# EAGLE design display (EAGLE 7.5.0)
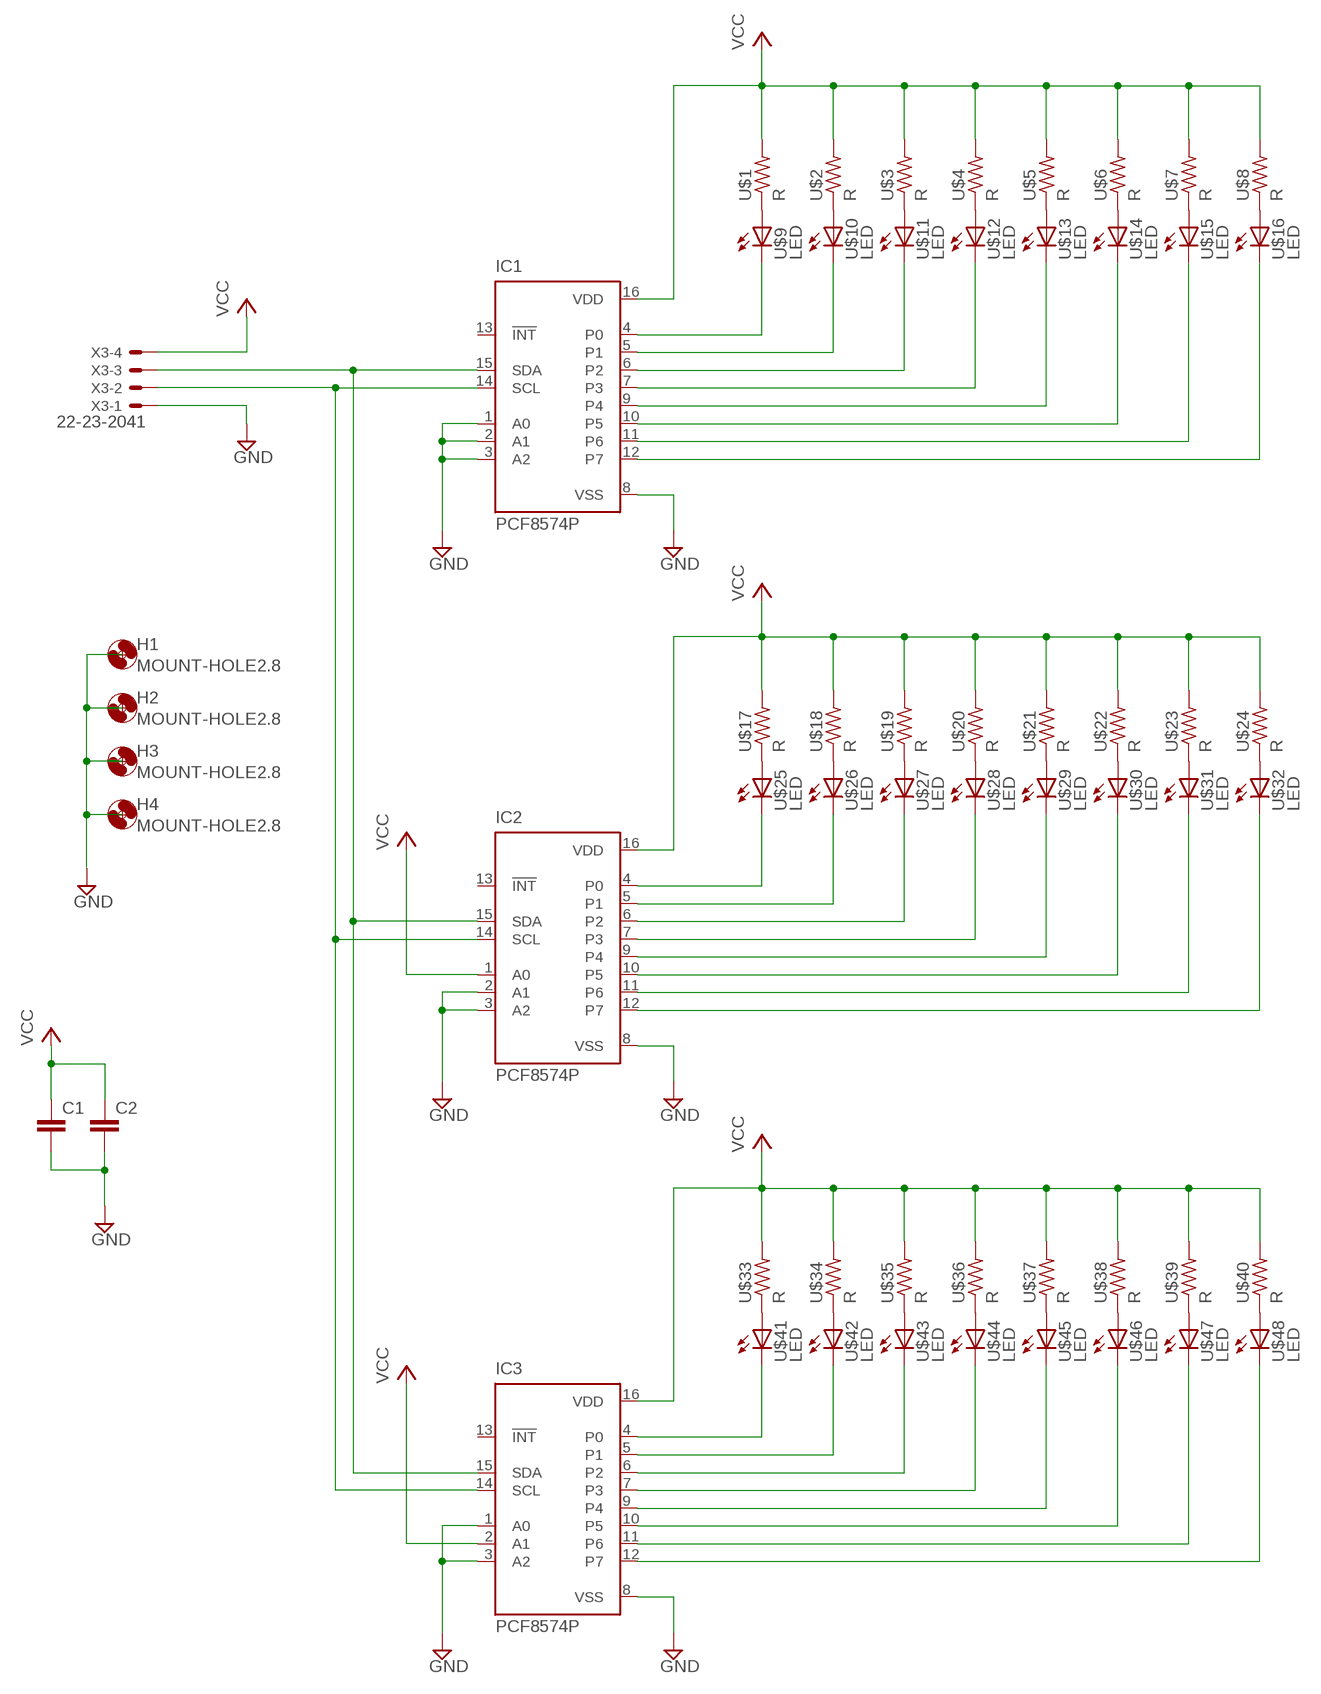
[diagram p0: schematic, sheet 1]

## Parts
C1  C-EU050-045X075  [C050-045X075]
C2  C-EU050-045X075  [C050-045X075]
H1  MOUNT-HOLE2.8  [2,8]
H2  MOUNT-HOLE2.8  [2,8]
H3  MOUNT-HOLE2.8  [2,8]
H4  MOUNT-HOLE2.8  [2,8]
IC1  PCF8574P  [DIL16]
IC2  PCF8574P  [DIL16]
IC3  PCF8574P  [DIL16]
U$1  R  [R]
U$2  R  [R]
U$3  R  [R]
U$4  R  [R]
U$5  R  [R]
U$6  R  [R]
U$7  R  [R]
U$8  R  [R]
U$9  LED  [LED]
U$10  LED  [LED]
U$11  LED  [LED]
U$12  LED  [LED]
U$13  LED  [LED]
U$14  LED  [LED]
U$15  LED  [LED]
U$16  LED  [LED]
U$17  R  [R]
U$18  R  [R]
U$19  R  [R]
U$20  R  [R]
U$21  R  [R]
U$22  R  [R]
U$23  R  [R]
U$24  R  [R]
U$25  LED  [LED]
U$26  LED  [LED]
U$27  LED  [LED]
U$28  LED  [LED]
U$29  LED  [LED]
U$30  LED  [LED]
U$31  LED  [LED]
U$32  LED  [LED]
U$33  R  [R]
U$34  R  [R]
U$35  R  [R]
U$36  R  [R]
U$37  R  [R]
U$38  R  [R]
U$39  R  [R]
U$40  R  [R]
U$41  LED  [LED]
U$42  LED  [LED]
U$43  LED  [LED]
U$44  LED  [LED]
U$45  LED  [LED]
U$46  LED  [LED]
U$47  LED  [LED]
U$48  LED  [LED]
X3  22-23-2041  [22-23-2041]

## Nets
GND: C1.2 C2.2 IC1.1(A0) IC1.2(A1) IC1.3(A2) IC1.8(VSS) IC2.2(A1) IC2.3(A2) IC2.8(VSS) IC3.1(A0) IC3.3(A2) IC3.8(VSS) X3.1
N$1: U$1.1 U$9.A
N$2: U$2.1 U$10.A
N$3: U$3.1 U$11.A
N$4: U$4.1 U$12.A
N$5: U$5.1 U$13.A
N$6: U$6.1 U$14.A
N$7: U$7.1 U$15.A
N$8: U$8.1 U$16.A
N$9: IC1.15(SDA) IC2.15(SDA) IC3.15(SDA) X3.3
N$10: IC1.4(P0) U$9.K(C)
N$11: IC1.5(P1) U$10.K(C)
N$12: IC1.6(P2) U$11.K(C)
N$13: IC1.7(P3) U$12.K(C)
N$14: IC1.9(P4) U$13.K(C)
N$15: IC1.10(P5) U$14.K(C)
N$16: IC1.11(P6) U$15.K(C)
N$17: IC1.12(P7) U$16.K(C)
N$18: U$17.1 U$25.A
N$19: U$18.1 U$26.A
N$20: U$19.1 U$27.A
N$21: U$20.1 U$28.A
N$22: U$21.1 U$29.A
N$23: U$22.1 U$30.A
N$24: U$23.1 U$31.A
N$25: U$24.1 U$32.A
N$26: IC2.4(P0) U$25.K(C)
N$27: IC2.5(P1) U$26.K(C)
N$28: IC2.6(P2) U$27.K(C)
N$29: IC2.7(P3) U$28.K(C)
N$30: IC2.9(P4) U$29.K(C)
N$31: IC2.10(P5) U$30.K(C)
N$32: IC2.11(P6) U$31.K(C)
N$33: IC2.12(P7) U$32.K(C)
N$34: U$33.1 U$41.A
N$35: U$34.1 U$42.A
N$36: U$35.1 U$43.A
N$37: U$36.1 U$44.A
N$38: U$37.1 U$45.A
N$39: U$38.1 U$46.A
N$40: U$39.1 U$47.A
N$41: U$40.1 U$48.A
N$42: IC3.4(P0) U$41.K(C)
N$43: IC3.5(P1) U$42.K(C)
N$44: IC3.6(P2) U$43.K(C)
N$45: IC3.7(P3) U$44.K(C)
N$46: IC3.9(P4) U$45.K(C)
N$47: IC3.10(P5) U$46.K(C)
N$48: IC3.11(P6) U$47.K(C)
N$49: IC3.12(P7) U$48.K(C)
N$50: IC1.14(SCL) IC2.14(SCL) IC3.14(SCL) X3.2
VCC: C1.1 C2.1 IC1.16(VDD) IC2.1(A0) IC2.16(VDD) IC3.2(A1) IC3.16(VDD) U$1.2 U$2.2 U$3.2 U$4.2 U$5.2 U$6.2 U$7.2 U$8.2 U$17.2 U$18.2 U$19.2 U$20.2 U$21.2 U$22.2 U$23.2 U$24.2 U$33.2 U$34.2 U$35.2 U$36.2 U$37.2 U$38.2 U$39.2 U$40.2 X3.4
Unconnected: IC1.13(!INT) IC2.13(!INT) IC3.13(!INT)

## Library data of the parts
C1 C2 = rcl:C-EU: CAPACITOR, European symbol
H1-H4 = holes:MOUNT-HOLE: MOUNTING HOLE with drill center marker
IC1-IC3 = micro-philips:PCF8574: I2C-Bus Remote 8-bit I/O expander http://www.semiconductors.philips.com/acrobat_download/datasheets/PCF8574_4.pdf; MPN: PCF8574PN; OC_FARNELL: 204020; OC_NEWARK: 11N8515
U$1-U$8 U$17-U$24 U$33-U$40 = micro-bit:R
U$9-U$16 U$25-U$32 U$41-U$48 = micro-bit:LED
X3 = con-molex:22-23-2041: .100" (2.54mm) Center Header - 4 Pin; MF: MOLEX; MPN: 22-23-2041; OC_FARNELL: 1462920; OC_NEWARK: 38C0355

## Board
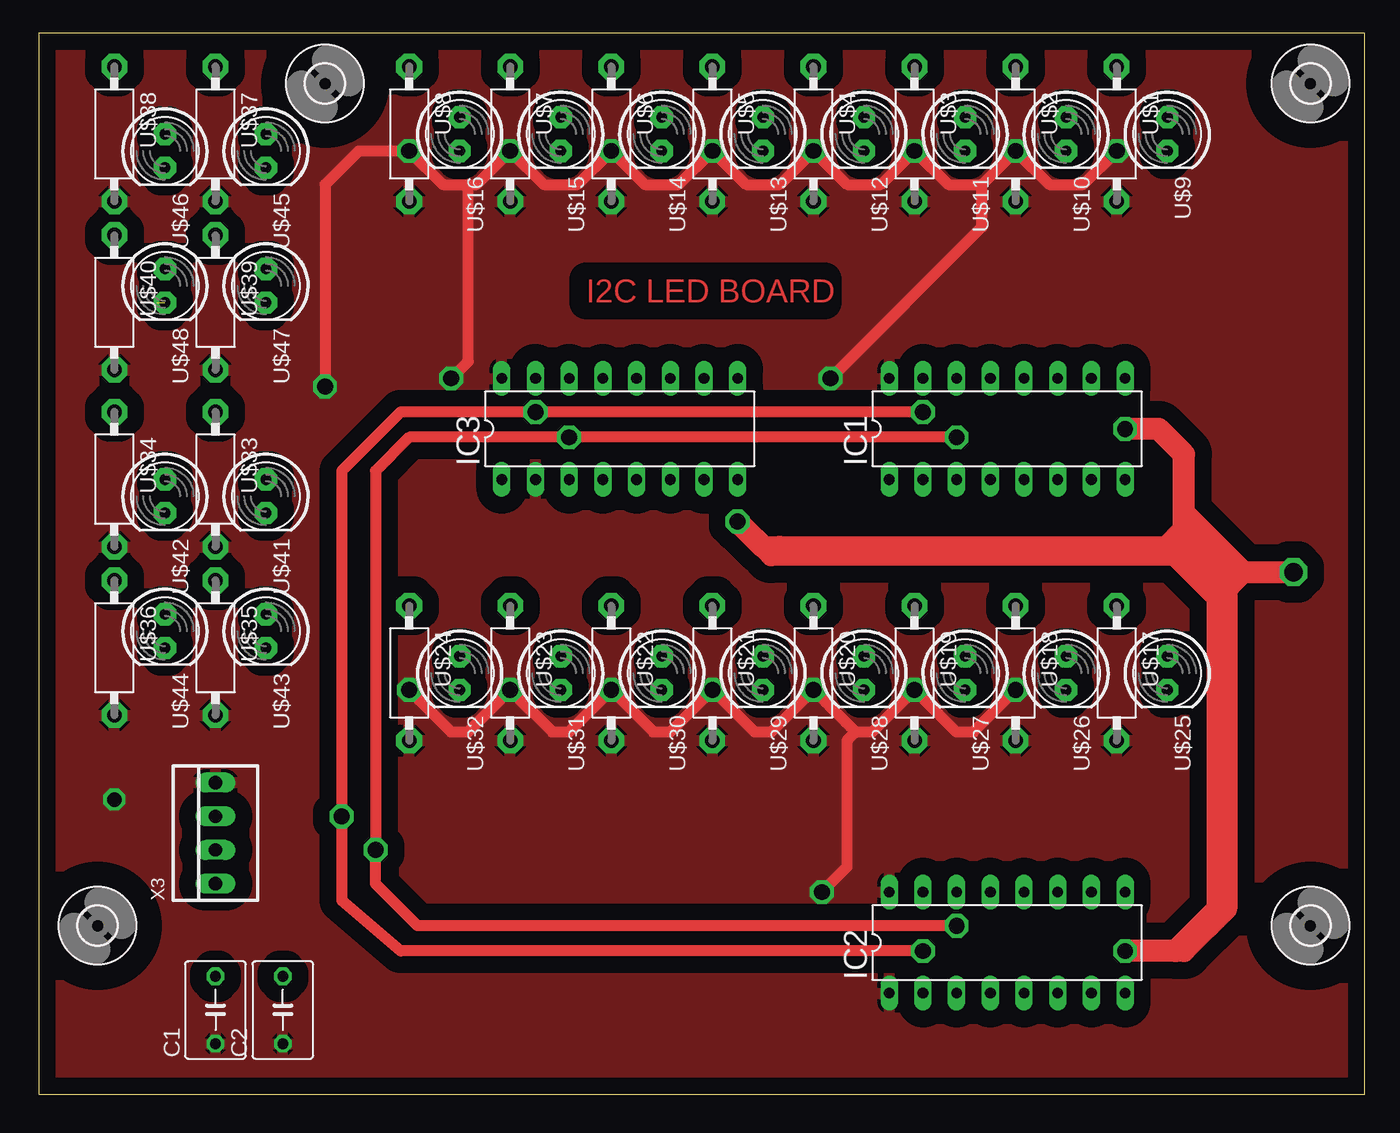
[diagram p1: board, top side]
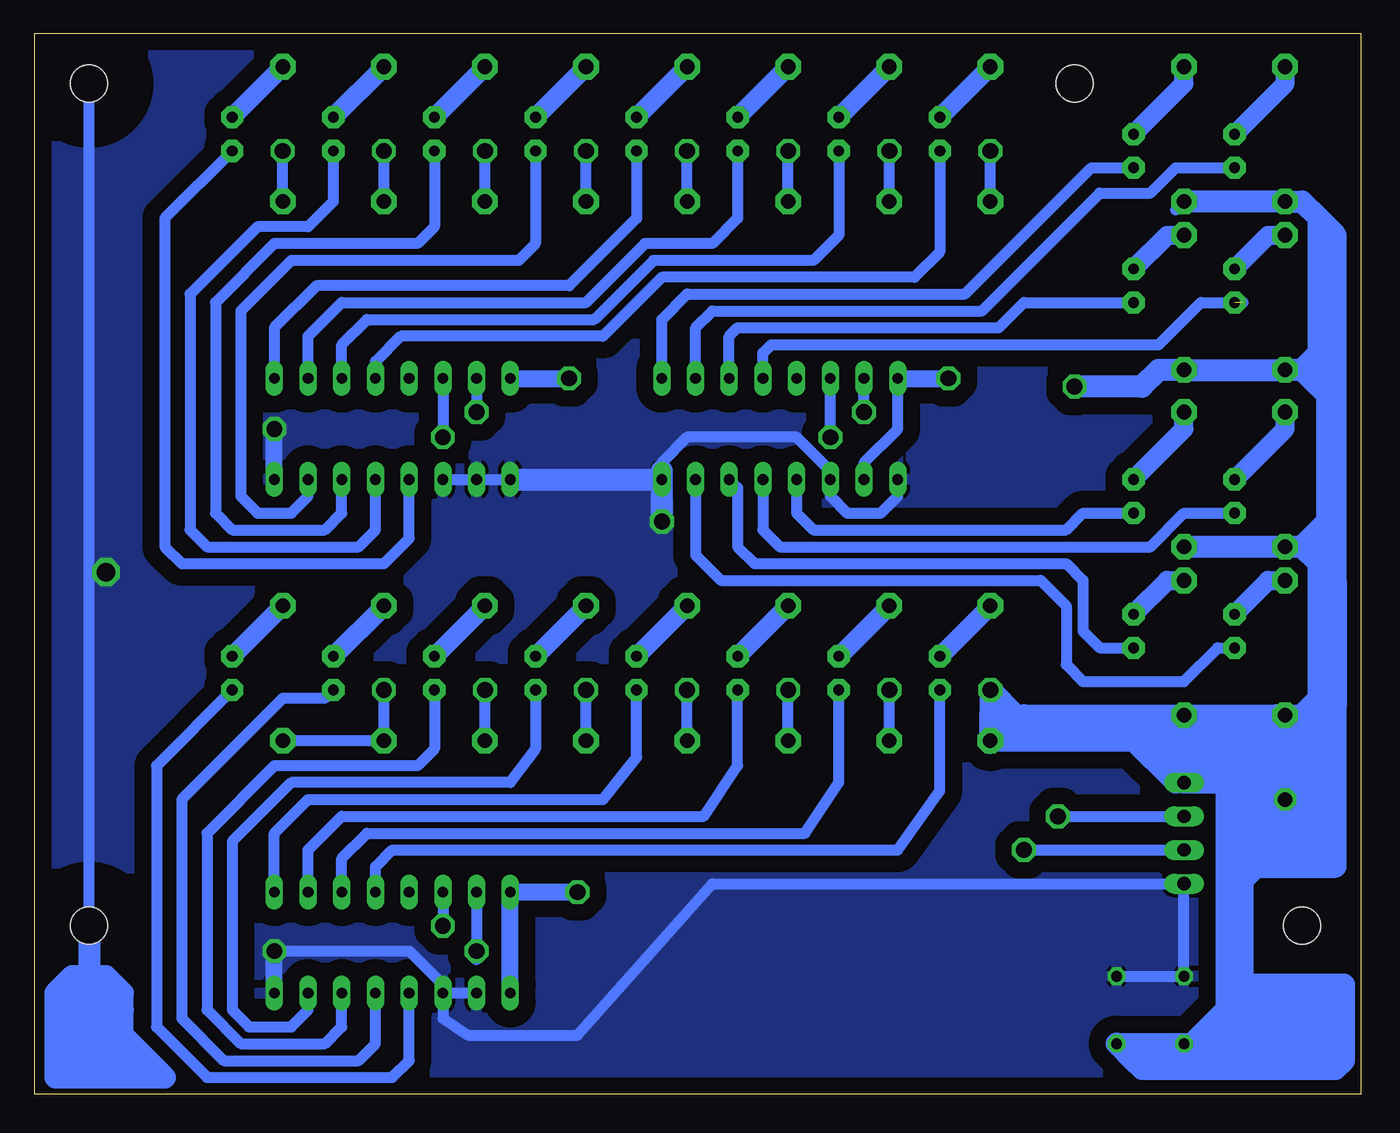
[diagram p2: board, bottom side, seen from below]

Size 100 x 80 mm. Coordinates in mm from the lower left corner, seen from the top.
Outline: 0,0 100,0 100,80 0,80 0,0
Copper layers (1*16): Top 0.035mm / dielectric 1.5mm / Bottom 0.035mm
Design rules "default": minimum track width 10mil, minimum drill 24mil, track to track 8mil, track to pad 8mil, pad to pad 8mil, via to via 8mil, smd to smd 8mil, copper to edge 40mil, drill to drill 8mil, minimum pad ring 10mil, minimum via ring 8mil, stop-mask expansion 4mil, vias tented up to drill 0mil, thermal gap 10mil

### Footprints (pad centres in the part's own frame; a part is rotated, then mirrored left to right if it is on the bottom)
C050-045X075 = drill 0.813 octagon: 1 -2.54,0; 2 2.54,0
2,8 = hole 2.8: 0,0
DIL16 = drill 0.813 long: 1 -8.89,-3.81; 2 -6.35,-3.81; 3 -3.81,-3.81; 4 -1.27,-3.81; 5 1.27,-3.81; 6 3.81,-3.81; 7 6.35,-3.81; 8 8.89,-3.81; 9 8.89,3.81; 10 6.35,3.81; 11 3.81,3.81; 12 1.27,3.81; 13 -1.27,3.81; 14 -3.81,3.81; 15 -6.35,3.81; 16 -8.89,3.81
R = drill 1.1 pad 1.93 octagon: 1 -5.08,0; 2 5.08,0
LED = drill 0.813 pad 1.676 octagon: A -1.27,0; K 1.27,0
22-23-2041 = drill 1 long: 1 -3.81,0; 2 -1.27,0; 3 1.27,0; 4 3.81,0

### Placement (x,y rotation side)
C1  13.34,6.35 90 top
C2  18.41,6.35 90 top
H1  4.45,12.7 0 top
H2  95.89,12.7 0 top
H3  95.89,76.2 0 top
H4  21.59,76.2 0 top
IC1  73.03,50.16 0 top
IC2  73.03,11.43 0 top
IC3  43.81,50.16 0 top
U$1  81.28,72.39 270 top
U$2  73.66,72.39 270 top
U$3  66.04,72.39 270 top
U$4  58.42,72.39 270 top
U$5  50.8,72.39 270 top
U$6  43.18,72.39 270 top
U$7  35.56,72.39 270 top
U$8  27.94,72.39 270 top
U$9  85.09,72.39 270 top
U$10  77.47,72.39 270 top
U$11  69.85,72.39 270 top
U$12  62.23,72.39 270 top
U$13  54.61,72.39 270 top
U$14  46.99,72.39 270 top
U$15  39.37,72.39 270 top
U$16  31.75,72.39 270 top
U$17  81.28,31.75 270 top
U$18  73.66,31.75 270 top
U$19  66.04,31.75 270 top
U$20  58.42,31.75 270 top
U$21  50.8,31.75 270 top
U$22  43.18,31.75 270 top
U$23  35.56,31.75 270 top
U$24  27.94,31.75 270 top
U$25  85.09,31.75 270 top
U$26  77.47,31.75 270 top
U$27  69.85,31.75 270 top
U$28  62.23,31.75 270 top
U$29  54.61,31.75 270 top
U$30  46.99,31.75 270 top
U$31  39.37,31.75 270 top
U$32  31.75,31.75 270 top
U$33  13.34,46.35 270 top
U$34  5.71,46.35 270 top
U$35  13.34,33.66 270 top
U$36  5.71,33.66 270 top
U$37  13.34,72.39 270 top
U$38  5.71,72.39 270 top
U$39  13.34,59.69 270 top
U$40  5.71,59.69 270 top
U$41  17.14,45.09 270 top
U$42  9.53,45.09 270 top
U$43  17.14,34.92 270 top
U$44  9.53,34.92 270 top
U$45  17.14,71.12 270 top
U$46  9.53,71.12 270 top
U$47  17.14,60.96 270 top
U$48  9.53,60.96 270 top
X3  13.34,19.68 90 top

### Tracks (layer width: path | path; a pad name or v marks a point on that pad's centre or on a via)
GND  (via drill 1.2 pad 0.41, 1.4)
  Top 0.813: 55.88,41.27 84.45,41.27 | 84.45,41.27 86.36,43.18 86.36,43.81 | 88.9,38.73 88.9,39.37 | 88.9,39.37 87,41.27 86.36,41.27 | 85.09,41.27 84.45,41.27 | 88.9,39.37 89.53,39.37
  Top 1.676: 85.09,41.27 55.88,41.27 54.61,41.27 v52.7,43.18 55.24,40.64 87,40.64 | 85.09,41.27 86.36,41.27 87,40.64 | 87,40.64 88.27,39.37 | 88.27,39.37 89.53,39.37 | 89.53,39.37 90.17,39.37 | 90.17,39.37 90.81,39.37 | 90.81,39.37 v94.61,39.37 | 85.09,41.27 86.36,42.55 | 86.36,43.81 86.36,48.26 84.45,50.16 v81.92,50.16 | 85.72,10.79 88.9,13.97 88.9,37.47 | 88.9,37.47 88.9,38.73 88.27,39.37 | 88.9,37.47 85.09,41.27 | 90.81,39.37 86.36,43.81 | 90.81,39.37 88.9,37.47 | 89.53,39.37 86.36,42.55 | 86.36,42.55 86.36,43.81 | 90.17,39.37 89.53,38.73 89.53,13.97 86.36,10.79 85.72,10.79 | 85.72,10.79 v81.92,10.79
  Bottom 0.813: IC2.8 v81.92,10.79 71.75,10.79 69.22,8.26 IC2.3 | IC1.1 IC1.2 IC1.3 | IC3.1 34.92,45.09 36.2,43.81 38.73,43.81 40.01,45.09 IC3.3 40.01,46.99 42.55,49.53 50.8,49.53 52.7,47.62 52.7,46.99 | IC2.2 IC2.3 | IC2.3 69.22,5.71 67.31,4.45 59.05,4.45 48.9,15.88 X3.1 C1.2 C2.2 | 95.89,12.7 95.89,39.37 | v94.61,39.37 95.89,39.37 | 95.89,39.37 95.89,76.2
  Bottom 1.27: IC1.8 v81.92,50.16 | 81.92,6.99 v81.92,10.79
  Bottom 1.676: IC1.1 IC3.8 | v52.7,43.18 IC3.8 | IC3.8 52.7,46.99
  pour Bottom (isolate 1.27): 0,80.01 100.33,80.01 100.33,0 62.23,0 18.41,0 0,0
N$1
  Bottom 1.422: U$9.A U$1.1
N$2
  Bottom 1.422: U$10.A U$2.1
N$3
  Bottom 1.422: U$11.A U$3.1
N$4
  Bottom 1.422: U$12.A U$4.1
N$5
  Bottom 1.422: U$13.A U$5.1
N$6
  Bottom 1.422: U$14.A U$6.1
N$7
  Bottom 1.422: U$15.A U$7.1
N$8
  Bottom 1.422: U$16.A U$8.1
N$9  (via drill 1.2 pad 0.41)
  Top 0.813: v66.67,51.44 v37.47,51.44 27.3,51.44 22.86,46.99 v22.86,20.95 22.86,14.61 27.3,10.79 v66.67,10.79
  Bottom 0.813: IC1.15 v66.67,51.44 | v37.47,51.44 IC3.15 | IC2.15 v66.67,10.79 66.67,10.16 | v22.86,20.95 X3.3
N$10
  Bottom 0.813: U$9.K 90.17,66.04 90.17,41.27 88.9,40.01 73.66,40.01 71.75,41.91 IC1.4
N$11
  Bottom 0.813: U$10.K 77.47,67.31 79.38,65.41 83.19,65.41 88.27,60.33 88.27,42.55 87,41.27 75.56,41.27 74.3,42.55 IC1.5
N$12
  Bottom 0.813: U$11.K 69.85,65.41 71.12,64.14 81.92,64.14 86.36,59.69 86.36,43.81 85.09,42.55 78.11,42.55 76.83,43.81 IC1.6
N$13
  Bottom 0.813: U$12.K 62.23,64.14 63.5,62.87 80.64,62.87 84.45,59.05 84.45,45.09 83.19,43.81 80.64,43.81 79.38,45.09 IC1.7
N$14
  Bottom 0.813: U$13.K 54.61,66.04 59.69,60.96 78.74,60.96 81.92,57.78 IC1.9
N$15
  Bottom 0.813: U$14.K 46.99,66.04 48.9,64.14 53.98,64.14 58.42,59.69 76.83,59.69 79.38,57.15 IC1.10
N$16
  Bottom 0.813: U$15.K 39.37,64.77 41.27,62.87 53.34,62.87 57.78,58.42 74.93,58.42 76.83,56.52 IC1.11
N$17
  Bottom 0.813: U$16.K 31.75,63.5 33.66,61.59 52.7,61.59 57.15,57.15 72.39,57.15 74.3,55.24 IC1.12
N$18
  Bottom 1.422: U$25.A U$17.1
N$19
  Bottom 1.422: U$26.A U$18.1
N$20
  Bottom 1.422: U$27.A U$19.1
N$21
  Bottom 1.422: U$28.A U$20.1
N$22
  Bottom 1.422: U$29.A U$21.1
N$23
  Bottom 1.422: U$30.A U$22.1
N$24
  Bottom 1.422: U$31.A U$23.1
N$25
  Bottom 1.422: U$32.A U$24.1
N$26
  Bottom 0.813: U$25.K 90.81,24.77 90.81,5.08 87,1.27 73.03,1.27 71.75,2.54 IC2.4
N$27
  Bottom 0.813: U$26.K 78.11,29.84 81.28,29.84 88.9,22.23 88.9,5.71 85.72,2.54 75.56,2.54 74.3,3.81 IC2.5
N$28
  Bottom 0.813: U$27.K 69.85,26.04 71.12,24.77 81.92,24.77 87,19.68 87,6.35 84.45,3.81 78.11,3.81 76.83,5.08 IC2.6
N$29
  Bottom 0.813: U$28.K 62.23,26.04 64.14,23.5 80.64,23.5 85.09,19.05 85.09,6.35 83.82,5.08 80.64,5.08 79.38,6.35 IC2.7
N$30
  Bottom 0.813: IC2.9 81.92,19.68 79.38,22.23 57.15,22.23 54.61,25.4 U$29.K
N$31
  Bottom 0.813: IC2.10 79.38,18.41 76.83,20.95 49.53,20.95 46.99,24.77 U$30.K
N$32
  Bottom 0.813: IC2.11 76.83,17.78 74.93,19.68 41.91,19.68 39.37,23.5 U$31.K
N$33
  Bottom 0.813: IC2.12 74.3,17.14 73.03,18.41 34.92,18.41 31.75,22.86 U$32.K
N$34
  Bottom 1.422: U$41.A 13.34,50.16 U$33.1
N$35
  Bottom 1.422: U$42.A 5.71,50.16 U$34.1
N$36
  Bottom 1.422: U$43.A 14.61,38.73 U$35.1
N$37
  Bottom 1.422: U$44.A 6.99,38.73 U$36.1
N$38
  Bottom 1.422: U$45.A 13.34,76.2 U$37.1
N$39
  Bottom 1.422: U$46.A 5.71,76.2 U$38.1
N$40
  Bottom 1.422: U$47.A 14.61,64.77 U$39.1
N$41
  Bottom 1.422: U$48.A 6.99,64.77 U$40.1
N$42
  Bottom 0.813: IC3.4 42.55,43.81 41.27,42.55 22.23,42.55 20.95,43.81 U$41.K
N$43
  Bottom 0.813: IC3.5 45.09,42.55 43.81,41.27 15.88,41.27 13.34,43.81 U$42.K
N$44
  Bottom 0.813: IC3.6 46.99,45.72 46.99,41.27 45.72,40.01 22.23,40.01 20.95,38.73 20.95,34.92 19.68,33.66 U$43.K
N$45
  Bottom 0.813: IC3.7 50.16,40.64 48.26,38.73 24.13,38.73 22.23,36.83 22.23,32.38 20.95,31.11 13.34,31.11 10.79,33.66 U$44.K
N$46
  Bottom 0.813: IC3.9 52.7,58.42 50.8,60.33 29.84,60.33 20.32,69.85 U$45.K
N$47
  Bottom 0.813: IC3.10 50.16,57.78 48.9,59.05 28.57,59.05 19.68,67.94 15.88,67.94 13.97,69.85 U$46.K
N$48
  Bottom 0.813: IC3.11 47.62,57.15 46.99,57.78 27.3,57.78 25.4,59.69 U$47.K
N$49  (1 unrouted)
  Bottom 0.813: IC3.12 45.09,55.88 44.45,56.52 15.24,56.52 12.06,59.69 8.89,59.69
N$50  (via drill 1.2 pad 0.41)
  Top 0.813: v69.22,49.53 v40.01,49.53 27.94,49.53 25.4,46.99 25.4,19.05 v25.4,18.41 25.4,15.88 28.57,12.7 v69.22,12.7
  Bottom 0.813: IC1.14 v69.22,49.53 | v40.01,49.53 IC3.14 | IC2.14 v69.22,12.7 | v25.4,18.41 X3.2
N$51
  Bottom 1.676: 95.89,12.06 95.89,8.89 | 95.89,8.89 95.89,1.91 | 95.89,8.89 98.42,6.35 | 98.42,6.35 98.42,5.71 98.42,1.27 91.44,1.27 | 91.44,1.27 93.34,3.17 93.34,6.35 | 93.34,6.35 94.61,7.62 | 95.89,8.89 94.61,7.62 | 94.61,7.62 94.61,5.08 | 94.61,5.08 94.61,2.54 93.98,1.91 93.34,1.91 93.98,2.54 97.16,2.54 96.52,3.17 96.52,6.35 97.79,5.08 97.79,3.81 | 91.44,1.27 90.17,1.27 93.98,5.08 94.61,5.08 | 93.34,6.35 93.34,7.62 94.61,8.89 97.16,8.89 98.42,7.62 98.42,6.35
N$52
  Bottom 1.676: 13.97,25.4 11.43,27.94
N$53
  Bottom 1.676: 2.54,38.73 2.54,55.88
VCC  (via drill 1.1, 1.2 pad 0.41)
  Top 0.813: v27.94,30.48 31.11,27.3 32.38,27.3 v35.56,30.48 38.73,27.3 40.01,27.3 v43.18,30.48 46.35,27.3 47.62,27.3 v50.8,30.48 53.98,27.3 55.24,27.3 v58.42,30.48 61.59,27.3 | 32.38,68.58 30.48,68.58 v27.94,71.12 24.13,71.12 21.59,68.58 v21.59,53.34 | 32.38,68.58 33.02,68.58 v35.56,71.12 38.1,68.58 40.64,68.58 v43.18,71.12 45.72,68.58 48.26,68.58 v50.8,71.12 53.34,68.58 55.88,68.58 v58.42,71.12 60.96,68.58 63.5,68.58 v66.04,71.12 68.58,68.58 71.12,68.58 | 71.12,68.58 v73.66,71.12 76.2,68.58 78.74,68.58 v81.28,71.12 | 61.59,27.3 62.87,27.3 v66.04,30.48 69.22,27.3 70.48,27.3 v73.66,30.48 | v31.11,53.98 32.38,55.24 32.38,68.58 | 61.59,27.3 60.96,26.67 60.96,17.14 v59.05,15.24 | v59.69,53.98 71.12,65.41 71.12,68.58
  Bottom 0.813: 27.94,26.04 U$24.2 | 4.45,41.27 U$34.2 U$33.2 | U$8.2 v27.94,71.12 | U$7.2 v35.56,71.12 | U$6.2 v43.18,71.12 | U$5.2 v50.8,71.12 | U$4.2 v58.42,71.12 | U$3.2 v66.04,71.12 | U$2.2 v73.66,71.12 | U$1.2 v81.28,71.12 | U$23.2 v35.56,30.48 | U$22.2 v43.18,30.48 | U$21.2 v50.8,30.48 | U$20.2 v58.42,30.48 | U$19.2 v66.04,30.48 | v73.66,30.48 U$18.2 U$17.2 | 25.4,28.57 27.3,28.57 | 27.3,28.57 27.94,27.94 U$24.2 | U$24.2 27.94,29.21 | v27.94,30.48 27.94,29.21 | 27.94,29.21 27.3,28.57 | U$37.2 13.97,66.67 | IC3.2 37.47,47.62 34.92,50.16 IC3.16 | C2.1 C1.1 12.7,3.81 10.79,3.81 8.89,3.81 8.89,5.71 8.89,8.26 | 8.89,24.77 8.89,26.04
  Bottom 1.27: 8.89,8.26 8.89,15.88 | 8.89,15.88 8.89,17.14 | 8.89,24.77 8.89,26.67 10.79,26.67 10.16,26.04 | 8.89,15.88 6.99,17.78 5.71,17.78 4.45,17.78 | v59.05,15.24 IC2.16 IC2.1 | IC1.16 v59.69,53.98 | IC3.16 v31.11,53.98
  Bottom 1.676: U$24.2 27.94,28.57 26.04,28.57 | 25.4,28.57 U$35.2 | U$24.2 v27.94,30.48 26.04,28.57 | U$24.2 27.3,26.67 26.67,27.3 | 26.67,27.3 25.4,28.57 | X3.4 13.34,24.77 | 13.34,24.77 13.34,25.4 | 13.34,25.4 13.34,27.3 | 13.34,27.3 U$35.2 | U$24.2 17.14,26.67 | 17.14,26.67 15.88,26.67 13.34,24.13 X3.4 | 13.34,25.4 14.61,26.67 14.61,27.3 26.67,27.3 | 26.04,28.57 25.4,28.57 | U$35.2 6.35,28.57 | 6.35,28.57 U$36.2 | U$36.2 6.99,27.3 13.34,27.3 | X3.4 10.16,26.67 8.89,26.67 7.62,26.67 6.35,27.94 6.35,28.57 | 13.34,24.77 11.43,26.67 | 4.45,54.61 3.17,55.88 3.17,66.04 | 3.17,66.04 4.45,67.31 U$38.2 U$37.2 | U$36.2 4.45,28.57 | 4.45,28.57 3.17,29.84 | 3.17,29.84 3.17,40.01 | 3.17,40.01 4.45,41.27 | 4.45,41.27 U$33.2 | v21.59,53.34 16.51,53.34 15.24,54.61 U$39.2 U$40.2 4.45,54.61 | 3.17,29.84 3.17,19.05 4.45,17.78 4.45,28.57 | 8.89,8.26 8.89,7.62 12.7,3.81 C2.1 17.14,2.54 | 8.89,17.14 8.89,24.77 10.16,26.04 | 10.16,26.04 11.43,26.04 | 17.14,2.54 16.51,1.91 1.91,1.91 1.27,2.54 1.27,8.26 8.89,8.26 | 8.89,8.26 8.89,17.14 | 8.89,17.14 1.91,17.14 1.91,29.21 | 1.91,29.21 3.17,27.94 3.17,17.78 | 3.17,40.01 1.91,38.73 | 1.91,38.73 1.91,29.21 | 5.71,27.94 v5.71,22.23 5.71,17.78 6.35,18.41 6.99,18.41 6.99,26.67 7.62,26.04 8.26,26.04 7.62,25.4 7.62,17.78 | 17.14,2.54 16.51,3.17 10.16,3.17 | 10.16,3.17 2.54,3.17 2.54,7.62 3.17,6.99 7.62,6.99 8.89,5.71 | 8.89,5.71 10.16,4.45 | 10.79,3.81 10.16,4.45 | 10.16,4.45 3.81,4.45 3.81,5.71 8.89,5.71 | 10.16,26.04 10.16,23.5 | 10.16,23.5 10.16,3.17 | X3.4 10.16,23.5 | 10.16,23.5 11.43,24.77 | X3.4 13.97,23.5 17.14,26.67 | 4.45,41.27 1.91,43.81 1.91,52.07 4.45,54.61 | 1.91,38.73 1.91,64.77 3.17,66.04
  pour Top (isolate 1.27): 0,80.01 100.33,80.01 100.33,13.97 100.33,0 0,0 0,60.33

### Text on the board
Top: I2C LED BOARD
